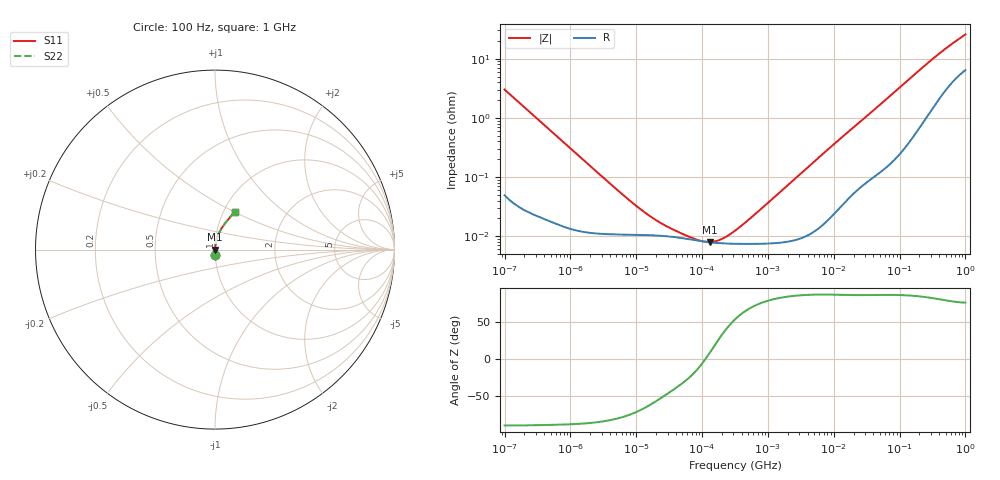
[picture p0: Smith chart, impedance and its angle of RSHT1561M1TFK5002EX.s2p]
! RSHT1561M1TFK5002EX  S-PARAMETER MODEL  (General Type)
! Model Generated by ELNA Corporation (http://www.ty-top.com)
! Version 1.0
! ELNA Control No.201201
! Copyright (c) 2020 ELNA CO.,LTD. All Rights Reserved.
! Products Name : CONDUCTIVE POLYMER HYBRID ALUMINUM ELECTROLYTIC CAPACITORS
! Characteristics :
!  Capacitance  :  560uF  ,  Rated voltage  :  25V
!  Operating Temp. Range  :  -55 to +105 degC  ,  Endurance  :  10000hr at 105 degC
!  Dimension D  :  10mm  ,  Dimension L  :  12.5mm
! Frequency Range : 100Hz - 1GHz
! External Node Assignments :
!  1  o---| |---o  2
# MHz S RI R 50
!Freq[MHz].  S11 Real  S11 Imag  S21 Real  S21 Imag  S12 Real  S12 Imag  S22 Real  S22 Imag
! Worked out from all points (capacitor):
!   401 points, 100 Hz to 1 GHz, reference 50 ohm
!   read as one part in series: C = 529 uF near 108 Hz
!   lowest |Z| = 7.98 mohm at 130.3 kHz (marker M1)
!   series resonance near 112.6 kHz, so ESL is about 3.8 nH
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0.0001  0.00139 -0.03  0.9986 0.03  0.9986 0.03  0.00139 -0.03
0.000113  0.00114 -0.0266  0.9989 0.0266  0.9989 0.0266  0.00114 -0.0266
0.000309  0.000315 -0.00976  0.9997 0.00976  0.9997 0.00976  0.000315 -0.00976
0.001488  0.000124 -0.00205  0.9999 0.00205  0.9999 0.00205  0.000124 -0.00205
0.008414  0.000106 -0.000365  0.9999 0.000365  0.9999 0.000365  0.000106 -0.000365
0.014207  0.000105 -0.000218  0.9999 0.000218  0.9999 0.000218  0.000105 -0.000218
0.022131  0.000102 -0.000141  0.9999 0.000141  0.9999 0.000141  0.000102 -0.000141
0.034475  9.8e-05 -9.05e-05  0.9999 9.05e-05  0.9999 9.05e-05  9.8e-05 -9.05e-05
0.05821  9.02e-05 -4.79e-05  0.9999 4.79e-05  0.9999 4.79e-05  9.02e-05 -4.79e-05
0.06569  8.82e-05 -3.91e-05  0.9999 3.91e-05  0.9999 3.91e-05  8.82e-05 -3.91e-05
0.130317  7.9e-05 1.13e-05  0.9999 -1.13e-05  0.9999 -1.13e-05  7.9e-05 1.13e-05
0.229087  7.54e-05 6.17e-05  0.9999 -6.17e-05  0.9999 -6.17e-05  7.54e-05 6.17e-05
0.258523  7.5e-05 7.48e-05  0.9999 -7.48e-05  0.9999 -7.48e-05  7.5e-05 7.48e-05
0.316228  7.45e-05 9.91e-05  0.9999 -9.91e-05  0.9999 -9.91e-05  7.45e-05 9.91e-05
0.679986  7.44e-05 0.000239  0.9999 -0.000239  0.9999 -0.000239  7.44e-05 0.000239
4.704354  0.000117 0.0017  0.9999 -0.0017  0.9999 -0.0017  0.000117 0.0017
11.88502  0.000306 0.00421  0.9997 -0.00421  0.9997 -0.00421  0.000306 0.00421
69.9842  0.00213 0.0228  0.9979 -0.0228  0.9979 -0.0228  0.00213 0.0228
163.1173  0.00752 0.0516  0.9925 -0.0516  0.9925 -0.0516  0.00752 0.0516
350.7519  0.0275 0.1023  0.9725 -0.1023  0.9725 -0.1023  0.0275 0.1023
616.595  0.0629 0.1551  0.9371 -0.1551  0.9371 -0.1551  0.0629 0.1551
1000  0.1087 0.2082  0.8913 -0.2082  0.8913 -0.2082  0.1087 0.2082
